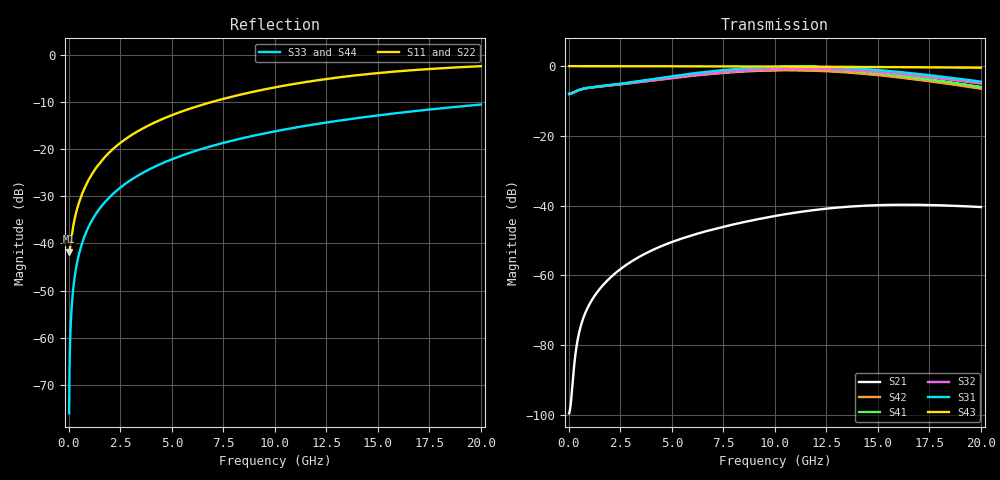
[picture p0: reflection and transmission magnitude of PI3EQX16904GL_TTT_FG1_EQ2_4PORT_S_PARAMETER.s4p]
! NPort=4 DATA=2000 NOISE=0 GROUPDELAY=0 COMPLEX_DATAFORMAT=POLAR
! NumOfBlock=1 NumOfParam=0
! .MODEL Smodel S TSTONEFILE=PI3EQX16904GL_TTT_FG1_EQ2_4PORT_S_PARAMETER.s4p TYPE=S
!  -- The above .MODEL line can be used for the S element in the netlist.
! The s parameter is extracted from the linear redriver, it is not bi-directional; only s(4,1)s(4,2) and s(3,1)s(3,2)
! should be the insertion loss
!Port definition:
!Port1 = input+
!Port2 = input-
!Port3 = output+
!Port4 = output-
# Hz S MA R  50
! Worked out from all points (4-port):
!   2000 points, 10 MHz to 20 GHz, reference 50 ohm
!   strongest paths, dB at 10 MHz, 5.01 GHz, 10.01 GHz, 15.01 GHz, 20 GHz:
!     S43: 0.0, 0.0, -0.1, -0.3, -0.4
!     S31: -8.0, -2.9, -0.2, -1.1, -4.4
!     S32: -8.0, -3.3, -0.8, -1.7, -5.0
!     S41: -8.0, -3.0, -0.6, -2.0, -5.9
!     S42: -8.0, -3.4, -1.2, -2.6, -6.5
!     S21: -99.6, -50.4, -43.0, -39.9, -40.4
!   lowest |S11| = -41.7 dB at 10 MHz (marker M1), VSWR 1.02, Z = 49.2 - j0.0603 ohm
!   |S11| at or under -10 dB: start of sweep to 6.906 GHz
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1e7  0.008182 -175.7  1.05e-05 7.6  0 0.0  0 0.0
     1.05e-05 7.6  0.008182 -175.7  0 0.0  0 0.0
     0.3995 0.2  0.3995 -179.8  0.0001571 -90.0  1 -0.0
     0.3995 -179.8  0.3995 0.2  1 -0.0  0.0001571 -90.0
2e8  0.01483 -130.6  3.383e-05 105.8  0 0.0  0 0.0
     3.383e-05 105.8  0.01483 -130.6  0 0.0  0 0.0
     0.4162 4.3  0.416 -175.9  0.003142 -90.2  1 -0.2
     0.4162 -176.0  0.416 3.7  1 -0.2  0.003142 -90.2
6.2e8  0.03268 -112.4  0.0002073 113.7  0 0.0  0 0.0
       0.0002073 113.7  0.03268 -112.4  0 0.0  0 0.0
       0.4688 4.1  0.4677 -176.5  0.009738 -90.6  0.9999 -0.6
       0.4688 -177.0  0.4677 2.4  0.9999 -0.6  0.009738 -90.6
2.97e9  0.1383 -101.6  0.001536 96.2  0 0.0  0 0.0
        0.001536 96.1  0.1384 -101.6  0 0.0  0 0.0
        0.5842 -11.2  0.5714 166.7  0.0466 -92.8  0.9988 -2.7
        0.5816 163.5  0.5689 -18.6  0.9988 -2.7  0.0466 -92.8
1.038e10  0.4707 -113.9  0.007492 42.5  0 0.0  0 0.0
          0.007419 42.7  0.4696 -114.0  0 0.0  0 0.0
          0.9881 -100.9  0.9197 78.6  0.1608 -99.6  0.9859 -9.3
          0.9376 61.1  0.8727 -119.4  0.9859 -9.3  0.1608 -99.6
1.463e10  0.6325 -124.2  0.01013 5.0  0 0.0  0 0.0
          0.01005 5.7  0.6307 -124.2  0 0.0  0 0.0
          0.8997 -163.9  0.8414 16.3  0.2235 -103.4  0.9726 -12.9
          0.8146 -8.5  0.7618 171.7  0.9726 -12.9  0.2235 -103.4
2e10  0.7628 -135.7  0.009571 -35.7  0 0.0  0 0.0
      0.009535 -34.7  0.7616 -135.6  0 0.0  0 0.0
      0.6003 125.6  0.5649 -53.8  0.2986 -108.1  0.9506 -17.4
      0.5054 -86.3  0.4756 94.3  0.9506 -17.4  0.2986 -108.1
